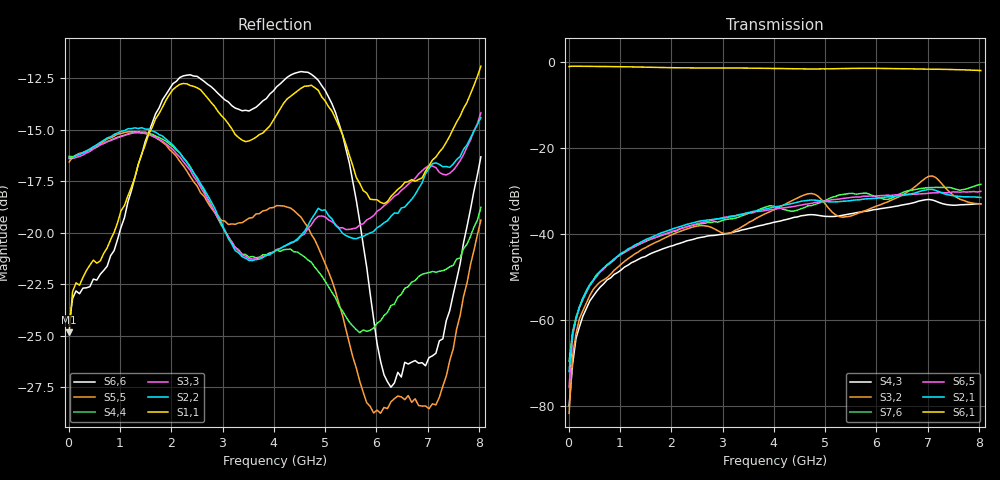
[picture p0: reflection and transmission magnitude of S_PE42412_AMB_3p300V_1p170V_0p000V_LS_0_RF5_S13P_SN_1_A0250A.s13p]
! Device ID: PE42412
! File Path: z:\PE42412\TE_GND_Post_Char_S-Param\All Parts\AMB\3p300\LS_0_RF5\PE42412_AMB_3p300V_1p170V_0p000V_LS_0_RF5_S13P_SN_1_A0250A.s13p
! Serial: 1
! Lot: A0250A
! Temp: AMB
! VDD: 3.300
! VSS: 0.000
! Control_Hi: 1.170
! Control_Lo: 0.000
! Logic State: LS_0_RF5
! Port 1:
! Port 2:
! Port 3:
! Port 4:
! Port 5:
! Port 6:
! Port 7:
! Port 8:
! Port 9:
! Port 10:
! Port 11:
! Port 12:
! Port 13:
! ThroughPath:1-6
! IDD: 0.0001064049
! ISS/IDD2: 3.57e-008
! IDMM3/IDD3: -2.636e-007
! Comment:
#  Hz  S  RI  R  50
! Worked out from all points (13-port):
!   120 points, 10 MHz to 8.037 GHz, reference 50 ohm
!   strongest paths, dB at 10 MHz, 2.034 GHz, 4.057 GHz, 6.08 GHz, 8.037 GHz:
!     S6,1: -1.1, -1.4, -1.5, -1.5, -2.0
!     S2,1: -71.9, -38.8, -33.6, -31.6, -31.5
!     S6,5: -75.6, -39.3, -34.1, -31.1, -30.1
!     S7,6: -69.5, -39.4, -33.7, -31.6, -28.4
!     S3,2: -81.6, -40.0, -34.0, -33.2, -33.0
!     S4,3: -79.9, -42.7, -37.1, -34.1, -33.0
!   lowest |S11| = -24.8 dB at 10 MHz (marker M1), VSWR 1.12, Z = 55.2 - j2.99 ohm
!   |S11| at or under -10 dB: start of sweep to end of sweep
